PROGRAM p05_ST_if
VAR
	preklopnik: BOOL;
	lucka: BOOL;
	tipka1: BOOL;
	tipka2: BOOL;
END_VAR

// Stavek IF
IF preklopnik = TRUE THEN
	lucka := TRUE;
END_IF

// Če pogoj ni resničen, lucka ne spremeni stanja, torej se
// stanje ohranja/pomni. Eksplicitno bi to zapisali:
IF preklopnik = TRUE THEN
	lucka := TRUE;
ELSE
	lucka := lucka;
END_IF

// Smo to želeli? Ali bi radi ob izklopu preklopnika
// ugasnili tudi lučko?
IF preklopnik THEN
	lucka := TRUE;
ELSE
	lucka := FALSE;
END_IF

// Ali za to sploh potrebujemo pogojni stavek? Ne ...
lucka := preklopnik;

// Če se le da, pogojne stavke nadomestimo z logičnimi izrazi
IF preklopnik THEN
	IF tipka1 THEN
		lucka := TRUE;
	ELSE 
		lucka := FALSE;
	END_IF
ELSE
	lucka := tipka2;
END_IF

// Enako kot:
lucka := (preklopnik AND tipka1) OR (NOT preklopnik AND tipka2);

END_PROGRAM
